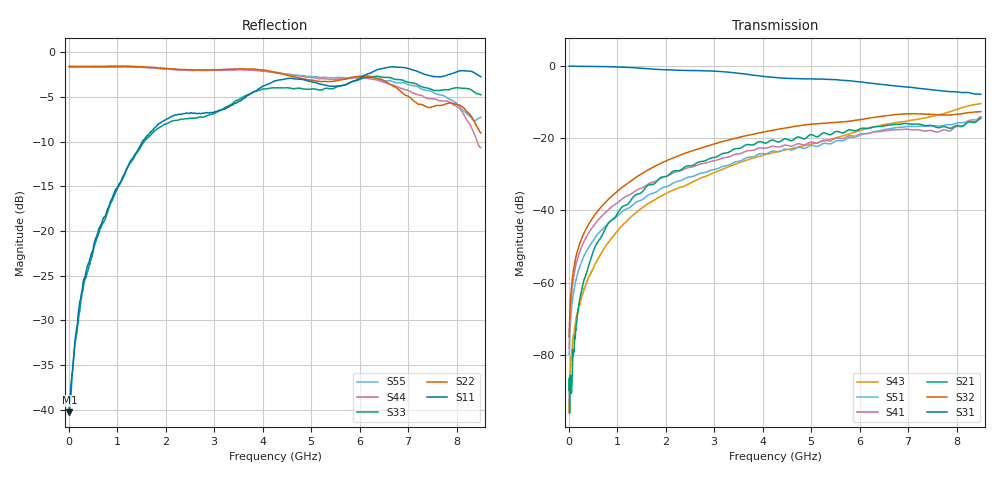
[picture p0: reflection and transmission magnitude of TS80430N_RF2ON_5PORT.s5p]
!Created with skrf (http://scikit-rf.org).
# GHz S RI R 50.0
!freq ReS11 ImS11 ReS12 ImS12 ReS13 ImS13
! ReS14 ImS14 ReS15 ImS15
! ReS21 ImS21 ReS22 ImS22 ReS23 ImS23
! ReS24 ImS24 ReS25 ImS25
! ReS31 ImS31 ReS32 ImS32 ReS33 ImS33
! ReS34 ImS34 ReS35 ImS35
! ReS41 ImS41 ReS42 ImS42 ReS43 ImS43
! ReS44 ImS44 ReS45 ImS45
! ReS51 ImS51 ReS52 ImS52 ReS53 ImS53
! ReS54 ImS54 ReS55 ImS55
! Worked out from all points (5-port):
!   1601 points, 10 MHz to 8.5 GHz, reference 50 ohm
!   strongest paths, dB at 10 MHz, 2.132 GHz, 4.255 GHz, 6.378 GHz, 8.5 GHz:
!     S31: -0.1, -1.2, -3.3, -5.1, -7.9
!     S32: -75.0, -25.6, -17.7, -14.1, -12.7
!     S21: -89.7, -29.3, -20.8, -16.8, -14.5
!     S41: -78.1, -29.8, -22.3, -18.2, -14.1
!     S51: -79.7, -32.6, -23.6, -18.0, -14.3
!     S43: -94.1, -34.5, -23.9, -16.6, -10.4
!   lowest |S11| = -40.3 dB at 15.31 MHz (marker M1), VSWR 1.02, Z = 50.9 - j0.338 ohm
!   |S11| at or under -10 dB: start of sweep to 1.52 GHz
